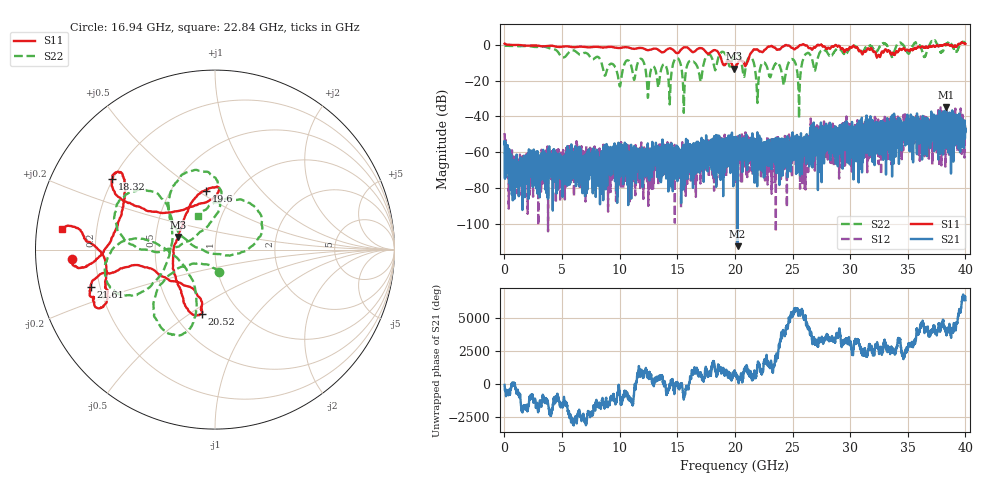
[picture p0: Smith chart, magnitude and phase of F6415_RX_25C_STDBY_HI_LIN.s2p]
!Keysight Technologies,N5245B,MY52451815,A.15.70.20
!Date: Wednesday, April 17, 2024 14:37:41
!Correction: S33(C  2-Port  )
!S43(C  2-Port  )
!S34(C  2-Port  )
!S44(C  2-Port  )
!S2P File: Measurements: S33, S43, S34, S44:
# Hz S  RI  R 50
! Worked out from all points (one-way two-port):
!   4000 points, 10 MHz to 40 GHz, reference 50 ohm
!   highest |S21| = -34.77 dB at 38.32 GHz (marker M1); lowest = -112.2 dB at 20.23 GHz (marker M2)
!   lowest |S11| = -13.3 dB at 19.94 GHz (marker M3), VSWR 1.55, Z = 32.8 + j4.79 ohm
!   |S11| at or under -10 dB: 18.9 GHz to 19.26 GHz (355.9 MHz wide, 1.87 % of centre); 19.67 GHz to 20.28 GHz (608.6 MHz wide, 3.05 % of centre); 20.77 GHz to 21.06 GHz (294.1 MHz wide, 1.41 % of centre)
!   |S22| runs from -41.1 to 2.3 dB; largest |S21 - S12| = 0.024
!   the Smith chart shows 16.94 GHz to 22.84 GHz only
!   S11 on the Smith chart (normalised r, x): 16.94 GHz: 0.11, -0.03; 18.32 GHz: 0.20, +0.30; 19.6 GHz: 0.73, +0.54; 20.52 GHz: 0.68, -0.56; 21.61 GHz: 0.16, -0.14; 22.84 GHz: 0.07, +0.07
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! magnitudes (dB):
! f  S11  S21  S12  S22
! 10 MHz  0.5  -55.5  -49.2  -0.7
! 1.36 GHz  -0.3  -74.3  -72.0  -0.9
! 6.68 GHz  -1.2  -66.1  -56.5  -5.4
! 13.34 GHz  -2.9  -64.8  -57.7  -23.9
! 14.94 GHz  -4.7  -60.2  -66.8  -7.3
! 15.55 GHz  -1.6  -59.0  -64.8  -34.3
! 16.12 GHz  -3.1  -67.7  -63.0  -9.0
! 16.94 GHz  -2.0  -56.9  -61.3  -17.9
! 18.32 GHz  -3.2  -54.9  -61.6  -13.9
! 19.6 GHz  -9.6  -50.6  -57.1  -11.8
! 19.94 GHz  -13.3  -52.7  -59.0  -5.4
! 20.01 GHz  -12.7  -58.9  -56.2  -4.9
! 20.23 GHz  -10.6  -112.2  -59.2  -4.8
! 20.52 GHz  -8.7  -52.7  -58.7  -8.6
! 21.61 GHz  -2.8  -58.4  -59.8  -9.6
! 22.84 GHz  -1.3  -67.4  -63.2  -13.6
! 25 GHz  -1.9  -48.8  -64.0  -8.2
! 25.56 GHz  -0.7  -60.6  -64.6  -41.1
! 26.67 GHz  -2.7  -50.8  -50.5  -7.6
! 33.34 GHz  -3.4  -49.9  -56.9  -2.0
! 38.32 GHz  -0.2  -34.8  -48.8  0.2
! 40 GHz  0.4  -46.8  -48.7  1.4
